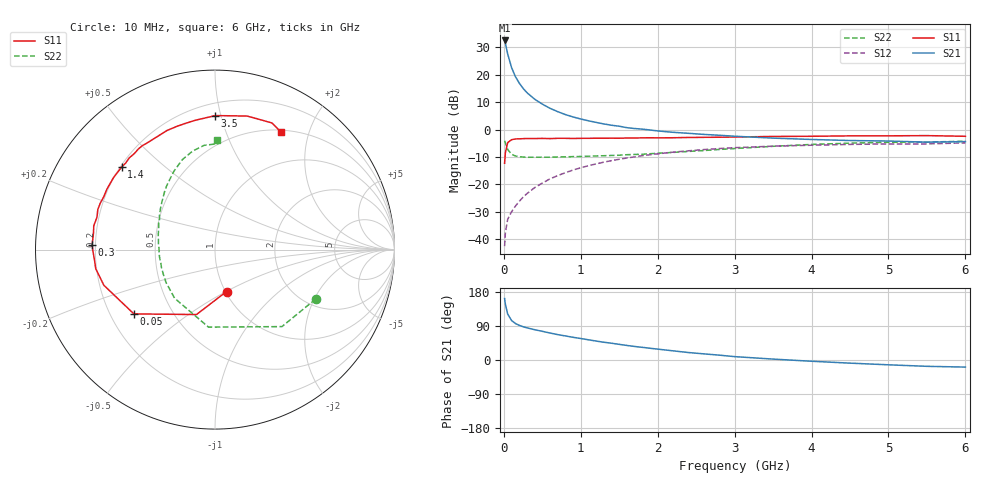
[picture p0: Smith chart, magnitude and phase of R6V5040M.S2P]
! SIEMENS Small Signal Semiconductors
! BFR193
! Si NPN RF Bipolar Junction Transistor in SOT23
! VCE = 0.5 V  IC = 40 mA
! Common Emitter S-Parameters:  May  1996
# GHz  S  MA  R  50
!  f  S11  S21  S12  S22
! GHz  MAG  ANG  MAG  ANG  MAG  ANG  MAG  ANG
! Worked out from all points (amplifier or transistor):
!   36 points, 10 MHz to 6 GHz, reference 50 ohm
!   highest |S21| = 32.5 dB at 10 MHz (marker M1)
!   |S21| within 3 dB of that: start of sweep to 35.05 MHz
!   unconditionally stable (mu >= 1): 194.2 MHz to end of sweep
!   at 250 MHz: K = 1.05, MAG = 18.5 dB, |S12| = -24.7 dB
!   at 1.4 GHz: K = 1.09, MAG = 4.6 dB, |S12| = -11.4 dB
!   at 6 GHz: K = 1.03, MAG = -0.8 dB, |S12| = -4.9 dB
!   S11 on the Smith chart (normalised r, x): 10 MHz: 1.01, -0.50; 50 MHz: 0.30, -0.32; 300 MHz: 0.19, +0.02; 1.4 GHz: 0.21, +0.36; 3.5 GHz: 0.28, +0.96; 6 GHz: 0.52, +1.58
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0.01  0.2422 -74.6  42.31 162.2  0.0074 70.3  0.6252 -26.1
0.02  0.3762 -105.9  37.5 147.2  0.0131 65.8  0.5684 -49.0
0.05  0.5767 -141.6  23.95 121.2  0.0229 53.4  0.4335 -94.8
0.1  0.6503 -162.2  13.58 104.4  0.0314 54.6  0.3522 -129.6
0.15  0.673 -170.9  9.266 96.3  0.0398 58.9  0.3289 -146.0
0.2  0.6746 -175.7  7.055 91.5  0.0487 62.8  0.3184 -155.2
0.25  0.681 -179.6  5.646 87.8  0.058 64.8  0.3145 -161.5
0.3  0.6848 177.7  4.715 84.9  0.0674 66.6  0.3111 -165.8
0.4  0.6831 172.4  3.583 80.0  0.0866 67.4  0.3119 -172.2
0.5  0.6883 168.9  2.91 75.7  0.1051 67.5  0.3117 -177.2
0.6  0.6818 164.6  2.438 71.2  0.1253 66.8  0.3119 179.4
0.7  0.6901 161.1  2.119 67.0  0.1439 65.9  0.3144 176.4
0.8  0.6897 158.1  1.873 63.5  0.1626 64.3  0.3171 173.4
1.1  0.6905 148.0  1.442 53.3  0.2182 59.5  0.3256 166.1
1.4  0.6941 138.5  1.197 44.3  0.2699 53.9  0.3358 159.3
1.7  0.699 129.8  1.042 35.7  0.3163 48.3  0.3504 152.4
2.2  0.707 117.0  0.889 24.2  0.3859 38.8  0.3817 142.6
3  0.7288 98.7  0.754 8.9  0.4657 24.1  0.4489 126.5
3.5  0.7467 89.9  0.696 2.4  0.4962 16.0  0.4935 117.6
4.5  0.7653 76.4  0.629 -8.3  0.5342 2.7  0.5634 102.7
5.5  0.7736 65.8  0.587 -16.7  0.5446 -9.1  0.5906 88.3
6  0.7517 60.9  0.601 -18.7  0.5702 -12.8  0.6101 89.0
